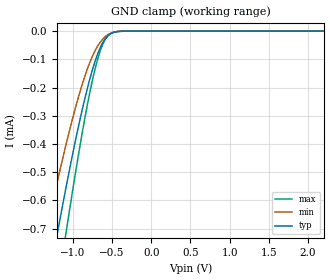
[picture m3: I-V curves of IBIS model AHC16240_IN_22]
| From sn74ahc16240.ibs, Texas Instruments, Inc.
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[Model]   AHC16240_IN_22
Model_type  Input
Vinl = 0.5
Vinh = 1.56
| variable   typ   min   max
C_comp   0.84pF   0.75pF   0.91pF
[Temperature Range]   40   100   -40
| Ambient temperature   25   85   -40
[Voltage range]   2.2   2   2.4
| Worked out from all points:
|   GND clamp passes 1 mA (typ) near -1.38 V on its own axis
[GND Clamp]
| AHC16240_IN_22
|   Voltage   I(typ)   I(min)   I(max)
-5.5V     -8.851mA   -7.354mA   -10.02mA
-1.355V   -959.3uA   -729.8uA   -1.218mA
-1.305V   -880.8uA   -665.9uA   -1.122mA
-1.205V   -727.2uA   -541.3uA   -931.7uA
-1.16V    -659.9uA   -487uA     -847.7uA
-1.09V    -557.7uA   -405.2uA   -719.4uA
-1.07V    -529.2uA   -382.5uA   -683.3uA
-895mV    -295.8uA   -201.7uA   -383.4uA
-745mV    -132.1uA   -85.68uA   -167uA
-635mV    -49.36uA   -33.72uA   -57.78uA
-530mV    -11.54uA   -9.155uA   -11.04uA
2.2V      580.3pA    219.9pA    1.028nA
